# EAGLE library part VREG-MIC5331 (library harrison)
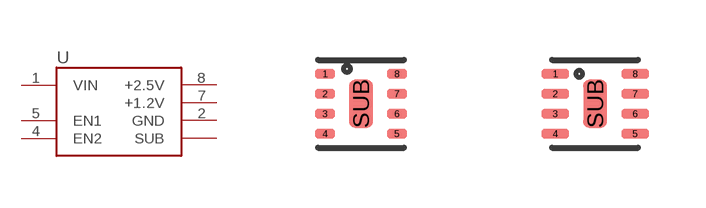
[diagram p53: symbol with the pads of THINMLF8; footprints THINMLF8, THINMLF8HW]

Designator prefix U

## VREG-MIC5331-J4YMT (RNUMBER: R00430; VAL: MIC5331-2.5/1.2)  [THINMLF8]
1  VIN  pwr
2  GND  pwr
4  EN2  in
5  EN1  in
7  +1.2V  pwr
8  +2.5V  pwr
SUB  SUB  pwr

## VREG-MIC5331-J4YMT-HW (RNUMBER: R00430; VAL: MIC5331-J4Y)  [THINMLF8HW]
Pads as for THINMLF8

## Footprint THINMLF8 (pad centres in mm)
smd 0.5 x 0.25: 1 -0.9,0.75; 2 -0.9,0.25; 3 -0.9,-0.25; 4 -0.9,-0.75; 5 0.9,-0.75; 6 0.9,-0.25; 7 0.9,0.25; 8 0.9,0.75
smd 0.6 x 1.2: SUB 0,0

## Footprint THINMLF8HW (pad centres in mm)
smd 0.7 x 0.25: 1 -1,0.75; 2 -1,0.25; 3 -1,-0.25; 4 -1,-0.75; 5 1,-0.75; 6 1,-0.25; 7 1,0.25; 8 1,0.75
smd 0.6 x 1.2: SUB 0,0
